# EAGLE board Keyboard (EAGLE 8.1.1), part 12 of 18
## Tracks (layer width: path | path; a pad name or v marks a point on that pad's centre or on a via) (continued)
S$12144 (continued)
  Bottom 0: 21.7,26.16 21.75,26.61
S$12145
  Bottom 0: 21.75,26.61 21.7,27.05
S$12146
  Bottom 0: 21.7,27.05 21.57,27.48
S$12147
  Bottom 0: 21.57,27.48 21.36,27.88
S$12148
  Bottom 0: 21.36,27.88 21.08,28.22
S$12149
  Bottom 0: 21.08,28.22 20.73,28.51
S$12150
  Bottom 0: 20.73,28.51 20.34,28.72
S$12151
  Bottom 0: 20.34,28.72 19.91,28.85
S$12152
  Bottom 0: 19.91,28.85 19.46,28.89
S$12153
  Bottom 0: 19.46,28.89 19.02,28.85
S$12154
  Bottom 0: 19.02,28.85 18.59,28.72
S$12155
  Bottom 0: 18.59,28.72 18.19,28.51
S$12156
  Bottom 0: 18.19,28.51 17.85,28.22
S$12157
  Bottom 0: 17.85,28.22 17.56,27.88
S$12158
  Bottom 0: 17.56,27.88 17.35,27.48
S$12159
  Bottom 0: 17.35,27.48 17.22,27.05
S$12160
  Bottom 0: 17.22,27.05 17.18,26.61
S$12161
  Bottom 0: 17.18,26.61 17.22,26.16
S$12162
  Bottom 0: 17.22,26.16 17.35,25.73
S$12163
  Bottom 0: 17.35,25.73 17.56,25.34
S$12164
  Bottom 0: 17.56,25.34 17.85,24.99
S$12165
  Bottom 0: 17.85,24.99 18.19,24.71
S$12166
  Bottom 0: 18.19,24.71 18.59,24.49
S$12167
  Bottom 0: 18.59,24.49 19.02,24.37
S$12168
  Bottom 0: 19.02,24.37 19.46,24.32
S$12169
  Bottom 0: 297.8,13.28 297.8,13.52
S$12170
  Bottom 0: 297.8,13.52 297.79,13.59
S$12171
  Bottom 0: 297.79,13.59 297.75,13.66
S$12172
  Bottom 0: 297.75,13.66 297.69,13.72
S$12173
  Bottom 0: 297.69,13.72 297.62,13.76
S$12174
  Bottom 0: 297.62,13.76 297.54,13.77
S$12175
  Bottom 0: 297.54,13.77 296.47,13.77
S$12176
  Bottom 0: 296.47,13.77 296.47,13.89
S$12177
  Bottom 0: 296.47,13.89 296.45,13.95
S$12178
  Bottom 0: 296.45,13.95 296.45,14
S$12179
  Bottom 0: 296.45,14 296.42,14.06
S$12180
  Bottom 0: 296.42,14.06 296.4,14.12
S$12181
  Bottom 0: 296.4,14.12 296.37,14.15
S$12182
  Bottom 0: 296.37,14.15 296.34,14.2
S$12183
  Bottom 0: 296.34,14.2 295.3,15.25
S$12184
  Bottom 0: 295.3,15.25 295.31,15.27
S$12185
  Bottom 0: 295.31,15.27 295.44,15.57
S$12186
  Bottom 0: 295.44,15.57 295.49,15.89
S$12187
  Bottom 0: 295.49,15.89 295.44,16.21
S$12188
  Bottom 0: 295.44,16.21 295.31,16.51
S$12189
  Bottom 0: 295.31,16.51 295.11,16.76
S$12190
  Bottom 0: 295.11,16.76 294.84,16.95
S$12191
  Bottom 0: 294.84,16.95 294.53,17.06
S$12192
  Bottom 0: 294.53,17.06 294.21,17.08
S$12193
  Bottom 0: 294.21,17.08 293.89,17.01
S$12194
  Bottom 0: 293.89,17.01 293.79,16.96
S$12195
  Bottom 0: 293.79,16.96 298.48,21.65
S$12196
  Bottom 0: 298.48,21.65 298.52,21.7
S$12197
  Bottom 0: 298.52,21.7 298.56,21.77
S$12198
  Bottom 0: 298.56,21.77 298.58,21.83
S$12199
  Bottom 0: 298.58,21.83 298.6,21.89
S$12200
  Bottom 0: 298.6,21.89 298.6,21.96
S$12201
  Bottom 0: 298.6,21.96 298.6,23.13
S$12202
  Bottom 0: 298.6,23.13 299.73,24.25
S$12203
  Bottom 0: 299.73,24.25 299.72,24.22
S$12204
  Bottom 0: 299.72,24.22 299.72,23.87
S$12205
  Bottom 0: 299.72,23.87 299.8,23.53
S$12206
  Bottom 0: 299.8,23.53 299.98,23.22
S$12207
  Bottom 0: 299.98,23.22 300.14,23.05
S$12208
  Bottom 0: 300.14,23.05 300.14,13.41
S$12209
  Bottom 0: 300.14,13.41 300.07,13.48
S$12210
  Bottom 0: 300.07,13.48 299.8,13.66
S$12211
  Bottom 0: 299.8,13.66 299.49,13.75
S$12212
  Bottom 0: 299.49,13.75 299.16,13.75
S$12213
  Bottom 0: 299.16,13.75 298.85,13.66
S$12214
  Bottom 0: 298.85,13.66 298.76,13.61
S$12215
  Bottom 0: 298.76,13.61 298.64,13.63
S$12216
  Bottom 0: 298.64,13.63 298.34,13.61
S$12217
  Bottom 0: 298.34,13.61 298.06,13.5
S$12218
  Bottom 0: 298.06,13.5 297.82,13.31
S$12219
  Bottom 0: 297.82,13.31 297.8,13.28
S$12220
  Bottom 0: 301.02,16.68 301.02,22.66
S$12221
  Bottom 0: 301.02,22.66 301.19,22.65
S$12222
  Bottom 0: 301.19,22.65 301.5,22.71
S$12223
  Bottom 0: 301.5,22.71 301.6,22.68
S$12224
  Bottom 0: 301.6,22.68 301.95,22.65
S$12225
  Bottom 0: 301.95,22.65 302.3,22.71
S$12226
  Bottom 0: 302.3,22.71 302.61,22.87
S$12227
  Bottom 0: 302.61,22.87 302.88,23.09
S$12228
  Bottom 0: 302.88,23.09 302.95,23.18
S$12229
  Bottom 0: 302.95,23.18 302.95,17.73
S$12230
  Bottom 0: 302.95,17.73 302.24,17.03
S$12231
  Bottom 0: 302.24,17.03 302.15,17.06
S$12232
  Bottom 0: 302.15,17.06 301.83,17.08
S$12233
  Bottom 0: 301.83,17.08 301.51,17.01
S$12234
  Bottom 0: 301.51,17.01 301.22,16.86
S$12235
  Bottom 0: 301.22,16.86 301.02,16.68
S$12236
  Bottom 0: 35.25,17.97 21.84,31.39
S$12237
  Bottom 0: 21.84,31.39 21.88,31.69
S$12238
  Bottom 0: 21.88,31.69 21.83,32.01
S$12239
  Bottom 0: 21.83,32.01 21.69,32.31
S$12240
  Bottom 0: 21.69,32.31 21.48,32.55
S$12241
  Bottom 0: 21.48,32.55 21.21,32.73
S$12242
  Bottom 0: 21.21,32.73 20.89,32.82
S$12243
  Bottom 0: 20.89,32.82 20.57,32.82
S$12244
  Bottom 0: 20.57,32.82 20.26,32.73
S$12245
  Bottom 0: 20.26,32.73 19.99,32.55
S$12246
  Bottom 0: 19.99,32.55 19.89,32.44
S$12247
  Bottom 0: 19.89,32.44 19.89,34.34
S$12248
  Bottom 0: 19.89,34.34 21.74,36.19
S$12249
  Bottom 0: 21.74,36.19 21.78,36.24
S$12250
  Bottom 0: 21.78,36.24 21.82,36.3
S$12251
  Bottom 0: 21.82,36.3 21.85,36.37
S$12252
  Bottom 0: 21.85,36.37 21.86,36.43
S$12253
  Bottom 0: 21.86,36.43 21.87,36.5
S$12254
  Bottom 0: 21.87,36.5 21.87,56.2
S$12255
  Bottom 0: 21.87,56.2 23.36,57.69
S$12256
  Bottom 0: 23.36,57.69 23.4,57.74
S$12257
  Bottom 0: 23.4,57.74 23.44,57.8
S$12258
  Bottom 0: 23.44,57.8 23.47,57.86
S$12259
  Bottom 0: 23.47,57.86 23.49,57.93
S$12260
  Bottom 0: 23.49,57.93 23.49,58
S$12261
  Bottom 0: 23.49,58 23.49,62.41
S$12262
  Bottom 0: 23.49,62.41 29.8,62.41
S$12263
  Bottom 0: 29.8,62.41 29.9,62.3
S$12264
  Bottom 0: 29.9,62.3 30.12,62.19
S$12265
  Bottom 0: 30.12,62.19 30.37,62.17
S$12266
  Bottom 0: 30.37,62.17 30.61,62.23
S$12267
  Bottom 0: 30.61,62.23 30.71,62.3
S$12268
  Bottom 0: 30.71,62.3 30.79,62.2
S$12269
  Bottom 0: 30.79,62.2 30.98,62
S$12270
  Bottom 0: 30.98,62 31.04,61.95
S$12271
  Bottom 0: 31.04,61.95 31.1,61.92
S$12272
  Bottom 0: 31.1,61.92 31.16,61.89
S$12273
  Bottom 0: 31.16,61.89 31.23,61.87
S$12274
  Bottom 0: 31.23,61.87 31.3,61.86
S$12275
  Bottom 0: 31.3,61.86 32.88,61.86
S$12276
  Bottom 0: 32.88,61.86 33.73,61.01
S$12277
  Bottom 0: 33.73,61.01 33.67,61.02
S$12278
  Bottom 0: 33.67,61.02 33.33,61
S$12279
  Bottom 0: 33.33,61 33,60.89
S$12280
  Bottom 0: 33,60.89 32.97,60.87
S$12281
  Bottom 0: 32.97,60.87 32.4,61.45
S$12282
  Bottom 0: 32.4,61.45 32.34,61.49
S$12283
  Bottom 0: 32.34,61.49 32.28,61.53
S$12284
  Bottom 0: 32.28,61.53 32.22,61.56
S$12285
  Bottom 0: 32.22,61.56 32.15,61.57
S$12286
  Bottom 0: 32.15,61.57 32.08,61.58
S$12287
  Bottom 0: 32.08,61.58 27.51,61.58
S$12288
  Bottom 0: 27.51,61.58 27.45,61.71
S$12289
  Bottom 0: 27.45,61.71 27.24,61.92
S$12290
  Bottom 0: 27.24,61.92 26.98,62.08
S$12291
  Bottom 0: 26.98,62.08 26.68,62.14
S$12292
  Bottom 0: 26.68,62.14 26.38,62.13
S$12293
  Bottom 0: 26.38,62.13 26.1,62.01
S$12294
  Bottom 0: 26.1,62.01 25.86,61.83
S$12295
  Bottom 0: 25.86,61.83 25.69,61.58
S$12296
  Bottom 0: 25.69,61.58 25.6,61.29
S$12297
  Bottom 0: 25.6,61.29 25.6,60.98
S$12298
  Bottom 0: 25.6,60.98 25.69,60.69
S$12299
  Bottom 0: 25.69,60.69 25.86,60.44
S$12300
  Bottom 0: 25.86,60.44 26.1,60.26
S$12301
  Bottom 0: 26.1,60.26 26.38,60.15
S$12302
  Bottom 0: 26.38,60.15 26.68,60.12
S$12303
  Bottom 0: 26.68,60.12 26.98,60.19
S$12304
  Bottom 0: 26.98,60.19 27.24,60.34
S$12305
  Bottom 0: 27.24,60.34 27.45,60.56
S$12306
  Bottom 0: 27.45,60.56 27.51,60.69
S$12307
  Bottom 0: 27.51,60.69 31.89,60.69
S$12308
  Bottom 0: 31.89,60.69 32.35,60.24
S$12309
  Bottom 0: 32.35,60.24 32.29,60.14
S$12310
  Bottom 0: 32.29,60.14 32.2,59.8
S$12311
  Bottom 0: 32.2,59.8 32.2,59.45
S$12312
  Bottom 0: 32.2,59.45 32.29,59.11
S$12313
  Bottom 0: 32.29,59.11 32.46,58.8
S$12314
  Bottom 0: 32.46,58.8 32.7,58.55
S$12315
  Bottom 0: 32.7,58.55 33,58.36
S$12316
  Bottom 0: 33,58.36 33.33,58.26
S$12317
  Bottom 0: 33.33,58.26 33.67,58.23
S$12318
  Bottom 0: 33.67,58.23 34.02,58.3
S$12319
  Bottom 0: 34.02,58.3 34.34,58.45
S$12320
  Bottom 0: 34.34,58.45 34.61,58.67
S$12321
  Bottom 0: 34.61,58.67 34.82,58.96
S$12322
  Bottom 0: 34.82,58.96 34.94,59.28
S$12323
  Bottom 0: 34.94,59.28 34.99,59.63
S$12324
  Bottom 0: 34.99,59.63 34.97,59.77
S$12325
  Bottom 0: 34.97,59.77 40.55,54.18
S$12326
  Bottom 0: 40.55,54.18 40.54,54.17
S$12327
  Bottom 0: 40.54,54.17 40.51,54.1
S$12328
  Bottom 0: 40.51,54.1 40.48,54.04
S$12329
  Bottom 0: 40.48,54.04 40.46,53.97
S$12330
  Bottom 0: 40.46,53.97 40.45,53.9
S$12331
  Bottom 0: 40.45,53.9 40.45,51.88
S$12332
  Bottom 0: 40.45,51.88 40.06,51.88
S$12333
  Bottom 0: 40.06,51.88 40.06,52.01
S$12334
  Bottom 0: 40.06,52.01 40,52.23
S$12335
  Bottom 0: 40,52.23 39.84,52.39
S$12336
  Bottom 0: 39.84,52.39 39.62,52.45
S$12337
  Bottom 0: 39.62,52.45 39.26,52.45
S$12338
  Bottom 0: 39.26,52.45 38.17,53.54
S$12339
  Bottom 0: 38.17,53.54 38.23,53.67
S$12340
  Bottom 0: 38.23,53.67 38.28,53.99
S$12341
  Bottom 0: 38.28,53.99 38.23,54.31
S$12342
  Bottom 0: 38.23,54.31 38.1,54.61
S$12343
  Bottom 0: 38.1,54.61 37.9,54.87
S$12344
  Bottom 0: 37.9,54.87 37.63,55.05
S$12345
  Bottom 0: 37.63,55.05 37.33,55.16
S$12346
  Bottom 0: 37.33,55.16 37.01,55.18
S$12347
  Bottom 0: 37.01,55.18 36.68,55.12
S$12348
  Bottom 0: 36.68,55.12 36.39,54.97
S$12349
  Bottom 0: 36.39,54.97 36.16,54.74
S$12350
  Bottom 0: 36.16,54.74 35.99,54.47
S$12351
  Bottom 0: 35.99,54.47 35.9,54.16
S$12352
  Bottom 0: 35.9,54.16 35.9,53.83
S$12353
  Bottom 0: 35.9,53.83 35.99,53.52
S$12354
  Bottom 0: 35.99,53.52 36.16,53.24
S$12355
  Bottom 0: 36.16,53.24 36.39,53.02
S$12356
  Bottom 0: 36.39,53.02 36.68,52.87
S$12357
  Bottom 0: 36.68,52.87 37.01,52.8
S$12358
  Bottom 0: 37.01,52.8 37.33,52.82
S$12359
  Bottom 0: 37.33,52.82 37.55,52.9
S$12360
  Bottom 0: 37.55,52.9 38.6,51.84
S$12361
  Bottom 0: 38.6,51.84 38.58,51.83
S$12362
  Bottom 0: 38.58,51.83 38.53,51.77
S$12363
  Bottom 0: 38.53,51.77 38.49,51.7
S$12364
  Bottom 0: 38.49,51.7 38.48,51.63
S$12365
  Bottom 0: 38.48,51.63 38.48,49.85
S$12366
  Bottom 0: 38.48,49.85 38.49,49.77
S$12367
  Bottom 0: 38.49,49.77 38.53,49.7
S$12368
  Bottom 0: 38.53,49.7 38.58,49.64
S$12369
  Bottom 0: 38.58,49.64 38.66,49.6
S$12370
  Bottom 0: 38.66,49.6 38.73,49.59
S$12371
  Bottom 0: 38.73,49.59 40.45,49.59
S$12372
  Bottom 0: 40.45,49.59 40.45,49.29
S$12373
  Bottom 0: 40.45,49.29 36.52,45.35
S$12374
  Bottom 0: 36.52,45.35 36.48,45.3
S$12375
  Bottom 0: 36.48,45.3 36.44,45.24
S$12376
  Bottom 0: 36.44,45.24 36.42,45.18
S$12377
  Bottom 0: 36.42,45.18 36.4,45.11
S$12378
  Bottom 0: 36.4,45.11 36.39,45.04
S$12379
  Bottom 0: 36.39,45.04 36.39,39.85
S$12380
  Bottom 0: 36.39,39.85 36.4,39.78
S$12381
  Bottom 0: 36.4,39.78 36.42,39.71
S$12382
  Bottom 0: 36.42,39.71 36.44,39.65
S$12383
  Bottom 0: 36.44,39.65 36.48,39.59
S$12384
  Bottom 0: 36.48,39.59 36.52,39.53
S$12385
  Bottom 0: 36.52,39.53 46.43,29.62
S$12386
  Bottom 0: 46.43,29.62 46.49,29.58
S$12387
  Bottom 0: 46.49,29.58 46.55,29.54
S$12388
  Bottom 0: 46.55,29.54 46.61,29.52
S$12389
  Bottom 0: 46.61,29.52 46.68,29.5
S$12390
  Bottom 0: 46.68,29.5 46.75,29.5
S$12391
  Bottom 0: 46.75,29.5 50.3,29.5
S$12392
  Bottom 0: 50.3,29.5 51,28.81
S$12393
  Bottom 0: 51,28.81 50.86,28.85
S$12394
  Bottom 0: 50.86,28.85 50.42,28.89
S$12395
  Bottom 0: 50.42,28.89 49.97,28.85
S$12396
  Bottom 0: 49.97,28.85 49.54,28.72
S$12397
  Bottom 0: 49.54,28.72 49.15,28.51
S$12398
  Bottom 0: 49.15,28.51 48.8,28.22
S$12399
  Bottom 0: 48.8,28.22 48.52,27.88
S$12400
  Bottom 0: 48.52,27.88 48.3,27.48
S$12401
  Bottom 0: 48.3,27.48 48.17,27.05
S$12402
  Bottom 0: 48.17,27.05 48.13,26.61
S$12403
  Bottom 0: 48.13,26.61 48.17,26.16
S$12404
  Bottom 0: 48.17,26.16 48.3,25.73
S$12405
  Bottom 0: 48.3,25.73 48.52,25.34
S$12406
  Bottom 0: 48.52,25.34 48.8,24.99
S$12407
  Bottom 0: 48.8,24.99 49.15,24.71
S$12408
  Bottom 0: 49.15,24.71 49.54,24.49
S$12409
  Bottom 0: 49.54,24.49 49.97,24.37
S$12410
  Bottom 0: 49.97,24.37 50.42,24.32
S$12411
  Bottom 0: 50.42,24.32 50.86,24.37
S$12412
  Bottom 0: 50.86,24.37 51.29,24.49
S$12413
  Bottom 0: 51.29,24.49 51.69,24.71
S$12414
  Bottom 0: 51.69,24.71 52.03,24.99
S$12415
  Bottom 0: 52.03,24.99 52.32,25.34
S$12416
  Bottom 0: 52.32,25.34 52.53,25.73
S$12417
  Bottom 0: 52.53,25.73 52.65,26.16
S$12418
  Bottom 0: 52.65,26.16 52.7,26.61
S$12419
  Bottom 0: 52.7,26.61 52.65,27.05
S$12420
  Bottom 0: 52.65,27.05 52.61,27.19
S$12421
  Bottom 0: 52.61,27.19 53.78,26.02
S$12422
  Bottom 0: 53.78,26.02 53.78,25.38
S$12423
  Bottom 0: 53.78,25.38 53.63,25.33
S$12424
  Bottom 0: 53.63,25.33 53.34,25.14
S$12425
  Bottom 0: 53.34,25.14 53.1,24.89
S$12426
  Bottom 0: 53.1,24.89 52.93,24.58
S$12427
  Bottom 0: 52.93,24.58 52.84,24.24
S$12428
  Bottom 0: 52.84,24.24 52.84,23.89
S$12429
  Bottom 0: 52.84,23.89 52.93,23.55
S$12430
  Bottom 0: 52.93,23.55 53.1,23.24
S$12431
  Bottom 0: 53.1,23.24 53.34,22.99
S$12432
  Bottom 0: 53.34,22.99 53.63,22.8
S$12433
  Bottom 0: 53.63,22.8 53.96,22.7
S$12434
  Bottom 0: 53.96,22.7 54.31,22.68
S$12435
  Bottom 0: 54.31,22.68 54.66,22.74
S$12436
  Bottom 0: 54.66,22.74 54.97,22.89
S$12437
  Bottom 0: 54.97,22.89 55.24,23.11
S$12438
  Bottom 0: 55.24,23.11 55.42,23.36
S$12439
  Bottom 0: 55.42,23.36 55.42,17.97
S$12440
  Bottom 0: 55.42,17.97 35.25,17.97
S$12441
  Bottom 0: 47.96,20.14 48.31,20.2
S$12442
  Bottom 0: 48.31,20.2 48.62,20.35
S$12443
  Bottom 0: 48.62,20.35 48.89,20.57
S$12444
  Bottom 0: 48.89,20.57 49.1,20.86
S$12445
  Bottom 0: 49.1,20.86 49.23,21.18
S$12446
  Bottom 0: 49.23,21.18 49.27,21.53
S$12447
  Bottom 0: 49.27,21.53 49.23,21.87
S$12448
  Bottom 0: 49.23,21.87 49.1,22.2
S$12449
  Bottom 0: 49.1,22.2 48.89,22.48
S$12450
  Bottom 0: 48.89,22.48 48.62,22.7
S$12451
  Bottom 0: 48.62,22.7 48.31,22.86
S$12452
  Bottom 0: 48.31,22.86 47.96,22.92
S$12453
  Bottom 0: 47.96,22.92 47.61,22.9
S$12454
  Bottom 0: 47.61,22.9 47.28,22.79
S$12455
  Bottom 0: 47.28,22.79 47.25,22.78
S$12456
  Bottom 0: 47.25,22.78 46.69,23.34
S$12457
  Bottom 0: 46.69,23.34 46.64,23.39
S$12458
  Bottom 0: 46.64,23.39 46.58,23.42
S$12459
  Bottom 0: 46.58,23.42 46.52,23.45
S$12460
  Bottom 0: 46.52,23.45 46.45,23.47
S$12461
  Bottom 0: 46.45,23.47 46.38,23.47
S$12462
  Bottom 0: 46.38,23.47 42.99,23.47
S$12463
  Bottom 0: 42.99,23.47 42.93,23.6
S$12464
  Bottom 0: 42.93,23.6 42.73,23.82
S$12465
  Bottom 0: 42.73,23.82 42.46,23.98
S$12466
  Bottom 0: 42.46,23.98 42.17,24.04
S$12467
  Bottom 0: 42.17,24.04 41.86,24.02
S$12468
  Bottom 0: 41.86,24.02 41.58,23.91
S$12469
  Bottom 0: 41.58,23.91 41.34,23.72
S$12470
  Bottom 0: 41.34,23.72 41.18,23.47
S$12471
  Bottom 0: 41.18,23.47 41.08,23.18
S$12472
  Bottom 0: 41.08,23.18 41.08,22.88
S$12473
  Bottom 0: 41.08,22.88 41.18,22.59
S$12474
  Bottom 0: 41.18,22.59 41.34,22.34
S$12475
  Bottom 0: 41.34,22.34 41.58,22.15
S$12476
  Bottom 0: 41.58,22.15 41.86,22.04
S$12477
  Bottom 0: 41.86,22.04 42.17,22.02
S$12478
  Bottom 0: 42.17,22.02 42.46,22.09
S$12479
  Bottom 0: 42.46,22.09 42.73,22.24
S$12480
  Bottom 0: 42.73,22.24 42.93,22.46
S$12481
  Bottom 0: 42.93,22.46 42.99,22.59
S$12482
  Bottom 0: 42.99,22.59 46.2,22.59
S$12483
  Bottom 0: 46.2,22.59 46.64,22.15
S$12484
  Bottom 0: 46.64,22.15 46.58,22.04
S$12485
  Bottom 0: 46.58,22.04 46.49,21.7
S$12486
  Bottom 0: 46.49,21.7 46.49,21.35
S$12487
  Bottom 0: 46.49,21.35 46.58,21.01
S$12488
  Bottom 0: 46.58,21.01 46.75,20.7
S$12489
  Bottom 0: 46.75,20.7 46.99,20.45
S$12490
  Bottom 0: 46.99,20.45 47.28,20.26
S$12491
  Bottom 0: 47.28,20.26 47.61,20.16
S$12492
  Bottom 0: 47.61,20.16 47.96,20.14
S$12493
  Bottom 0: 39.78,22.02 40.08,22.09
S$12494
  Bottom 0: 40.08,22.09 40.34,22.24
S$12495
  Bottom 0: 40.34,22.24 40.55,22.46
S$12496
  Bottom 0: 40.55,22.46 40.68,22.74
S$12497
  Bottom 0: 40.68,22.74 40.72,23.04
S$12498
  Bottom 0: 40.72,23.04 40.68,23.34
S$12499
  Bottom 0: 40.68,23.34 40.55,23.61
S$12500
  Bottom 0: 40.55,23.61 40.34,23.83
S$12501
  Bottom 0: 40.34,23.83 40.08,23.98
S$12502
  Bottom 0: 40.08,23.98 39.78,24.05
S$12503
  Bottom 0: 39.78,24.05 39.48,24.03
S$12504
  Bottom 0: 39.48,24.03 39.2,23.91
S$12505
  Bottom 0: 39.2,23.91 38.96,23.73
S$12506
  Bottom 0: 38.96,23.73 38.79,23.48
S$12507
  Bottom 0: 38.79,23.48 38.7,23.19
S$12508
  Bottom 0: 38.7,23.19 38.7,22.88
S$12509
  Bottom 0: 38.7,22.88 38.79,22.59
S$12510
  Bottom 0: 38.79,22.59 38.96,22.34
S$12511
  Bottom 0: 38.96,22.34 39.2,22.16
S$12512
  Bottom 0: 39.2,22.16 39.48,22.05
S$12513
  Bottom 0: 39.48,22.05 39.78,22.02
S$12514
  Bottom 0: 42.17,29.64 42.46,29.7
S$12515
  Bottom 0: 42.46,29.7 42.73,29.86
S$12516
  Bottom 0: 42.73,29.86 42.93,30.08
S$12517
  Bottom 0: 42.93,30.08 43.06,30.35
S$12518
  Bottom 0: 43.06,30.35 43.11,30.65
S$12519
  Bottom 0: 43.11,30.65 43.06,30.95
S$12520
  Bottom 0: 43.06,30.95 42.93,31.22
S$12521
  Bottom 0: 42.93,31.22 42.73,31.44
S$12522
  Bottom 0: 42.73,31.44 42.46,31.59
S$12523
  Bottom 0: 42.46,31.59 42.17,31.66
S$12524
  Bottom 0: 42.17,31.66 41.86,31.64
S$12525
  Bottom 0: 41.86,31.64 41.58,31.53
S$12526
  Bottom 0: 41.58,31.53 41.34,31.34
S$12527
  Bottom 0: 41.34,31.34 41.18,31.09
S$12528
  Bottom 0: 41.18,31.09 41.08,30.8
S$12529
  Bottom 0: 41.08,30.8 41.08,30.5
S$12530
  Bottom 0: 41.08,30.5 41.18,30.21
S$12531
  Bottom 0: 41.18,30.21 41.34,29.96
S$12532
  Bottom 0: 41.34,29.96 41.58,29.77
S$12533
  Bottom 0: 41.58,29.77 41.86,29.66
S$12534
  Bottom 0: 41.86,29.66 42.17,29.64
S$12535
  Bottom 0: 39.78,29.64 40.08,29.71
S$12536
  Bottom 0: 40.08,29.71 40.34,29.86
S$12537
  Bottom 0: 40.34,29.86 40.55,30.08
S$12538
  Bottom 0: 40.55,30.08 40.68,30.36
S$12539
  Bottom 0: 40.68,30.36 40.72,30.66
S$12540
  Bottom 0: 40.72,30.66 40.68,30.95
S$12541
  Bottom 0: 40.68,30.95 40.55,31.23
S$12542
  Bottom 0: 40.55,31.23 40.34,31.45
S$12543
  Bottom 0: 40.34,31.45 40.08,31.6
S$12544
  Bottom 0: 40.08,31.6 39.78,31.67
S$12545
  Bottom 0: 39.78,31.67 39.48,31.65
S$12546
  Bottom 0: 39.48,31.65 39.2,31.53
S$12547
  Bottom 0: 39.2,31.53 38.96,31.35
S$12548
  Bottom 0: 38.96,31.35 38.79,31.1
S$12549
  Bottom 0: 38.79,31.1 38.7,30.81
S$12550
  Bottom 0: 38.7,30.81 38.7,30.5
S$12551
  Bottom 0: 38.7,30.5 38.79,30.21
S$12552
  Bottom 0: 38.79,30.21 38.96,29.96
S$12553
  Bottom 0: 38.96,29.96 39.2,29.78
S$12554
  Bottom 0: 39.2,29.78 39.48,29.66
S$12555
  Bottom 0: 39.48,29.66 39.78,29.64
S$12556
  Bottom 0: 32.64,35.12 32.94,35.18
S$12557
  Bottom 0: 32.94,35.18 33.2,35.33
S$12558
  Bottom 0: 33.2,35.33 33.4,35.55
S$12559
  Bottom 0: 33.4,35.55 33.53,35.83
S$12560
  Bottom 0: 33.53,35.83 33.58,36.13
S$12561
  Bottom 0: 33.58,36.13 33.53,36.43
S$12562
  Bottom 0: 33.53,36.43 33.4,36.7
S$12563
  Bottom 0: 33.4,36.7 33.2,36.92
S$12564
  Bottom 0: 33.2,36.92 32.94,37.07
S$12565
  Bottom 0: 32.94,37.07 32.64,37.14
S$12566
  Bottom 0: 32.64,37.14 32.34,37.12
S$12567
  Bottom 0: 32.34,37.12 32.05,37.01
S$12568
  Bottom 0: 32.05,37.01 31.82,36.82
S$12569
  Bottom 0: 31.82,36.82 31.65,36.57
S$12570
  Bottom 0: 31.65,36.57 31.56,36.28
S$12571
  Bottom 0: 31.56,36.28 31.56,35.97
S$12572
  Bottom 0: 31.56,35.97 31.65,35.68
S$12573
  Bottom 0: 31.65,35.68 31.82,35.44
S$12574
  Bottom 0: 31.82,35.44 32.05,35.25
S$12575
  Bottom 0: 32.05,35.25 32.34,35.14
S$12576
  Bottom 0: 32.34,35.14 32.64,35.12
S$12577
  Bottom 0: 23.11,35.12 23.4,35.18
S$12578
  Bottom 0: 23.4,35.18 23.67,35.33
S$12579
  Bottom 0: 23.67,35.33 23.87,35.55
S$12580
  Bottom 0: 23.87,35.55 24.01,35.83
S$12581
  Bottom 0: 24.01,35.83 24.05,36.13
S$12582
  Bottom 0: 24.05,36.13 24.01,36.43
S$12583
  Bottom 0: 24.01,36.43 23.87,36.7
S$12584
  Bottom 0: 23.87,36.7 23.67,36.92
S$12585
  Bottom 0: 23.67,36.92 23.4,37.07
S$12586
  Bottom 0: 23.4,37.07 23.11,37.14
S$12587
  Bottom 0: 23.11,37.14 22.81,37.12
S$12588
  Bottom 0: 22.81,37.12 22.53,37.01
S$12589
  Bottom 0: 22.53,37.01 22.29,36.82
S$12590
  Bottom 0: 22.29,36.82 22.12,36.57
S$12591
  Bottom 0: 22.12,36.57 22.03,36.28
S$12592
  Bottom 0: 22.03,36.28 22.03,35.97
S$12593
  Bottom 0: 22.03,35.97 22.12,35.68
S$12594
  Bottom 0: 22.12,35.68 22.29,35.44
S$12595
  Bottom 0: 22.29,35.44 22.53,35.25
S$12596
  Bottom 0: 22.53,35.25 22.81,35.14
S$12597
  Bottom 0: 22.81,35.14 23.11,35.12
S$12598
  Bottom 0: 32.64,42.74 32.94,42.8
S$12599
  Bottom 0: 32.94,42.8 33.2,42.95
S$12600
  Bottom 0: 33.2,42.95 33.4,43.17
S$12601
  Bottom 0: 33.4,43.17 33.53,43.44
S$12602
  Bottom 0: 33.53,43.44 33.58,43.75
S$12603
  Bottom 0: 33.58,43.75 33.53,44.05
S$12604
  Bottom 0: 33.53,44.05 33.4,44.32
S$12605
  Bottom 0: 33.4,44.32 33.2,44.54
S$12606
  Bottom 0: 33.2,44.54 32.94,44.69
S$12607
  Bottom 0: 32.94,44.69 32.64,44.76
S$12608
  Bottom 0: 32.64,44.76 32.34,44.74
S$12609
  Bottom 0: 32.34,44.74 32.05,44.62
S$12610
  Bottom 0: 32.05,44.62 31.82,44.44
S$12611
  Bottom 0: 31.82,44.44 31.65,44.19
S$12612
  Bottom 0: 31.65,44.19 31.56,43.9
S$12613
  Bottom 0: 31.56,43.9 31.56,43.59
S$12614
  Bottom 0: 31.56,43.59 31.65,43.3
S$12615
  Bottom 0: 31.65,43.3 31.82,43.06
S$12616
  Bottom 0: 31.82,43.06 32.05,42.87
S$12617
  Bottom 0: 32.05,42.87 32.34,42.75
S$12618
  Bottom 0: 32.34,42.75 32.64,42.74
S$12619
  Bottom 0: 23.11,42.74 23.4,42.8
S$12620
  Bottom 0: 23.4,42.8 23.67,42.95
S$12621
  Bottom 0: 23.67,42.95 23.87,43.17
S$12622
  Bottom 0: 23.87,43.17 24.01,43.44
S$12623
  Bottom 0: 24.01,43.44 24.05,43.75
S$12624
  Bottom 0: 24.05,43.75 24.01,44.05
S$12625
  Bottom 0: 24.01,44.05 23.87,44.32
S$12626
  Bottom 0: 23.87,44.32 23.67,44.54
S$12627
  Bottom 0: 23.67,44.54 23.4,44.69
S$12628
  Bottom 0: 23.4,44.69 23.11,44.76
S$12629
  Bottom 0: 23.11,44.76 22.81,44.74
S$12630
  Bottom 0: 22.81,44.74 22.53,44.62
S$12631
  Bottom 0: 22.53,44.62 22.29,44.44
S$12632
  Bottom 0: 22.29,44.44 22.12,44.19
S$12633
  Bottom 0: 22.12,44.19 22.03,43.9
S$12634
  Bottom 0: 22.03,43.9 22.03,43.59
S$12635
  Bottom 0: 22.03,43.59 22.12,43.3
S$12636
  Bottom 0: 22.12,43.3 22.29,43.06
S$12637
  Bottom 0: 22.29,43.06 22.53,42.87
S$12638
  Bottom 0: 22.53,42.87 22.81,42.75
S$12639
  Bottom 0: 22.81,42.75 23.11,42.74
S$12640
  Bottom 0: 29.33,43.59 29.68,43.79
S$12641
  Bottom 0: 29.68,43.79 30.09,44.13
S$12642
  Bottom 0: 30.09,44.13 30.45,44.53
S$12643
  Bottom 0: 30.45,44.53 30.73,44.97
S$12644
  Bottom 0: 30.73,44.97 30.74,44.99
S$12645
  Bottom 0: 30.74,44.99 29.33,44.99
S$12646
  Bottom 0: 29.33,44.99 29.33,43.59
S$12647
  Bottom 0: 26.28,43.59 26.28,44.99
S$12648
  Bottom 0: 26.28,44.99 24.89,44.99
S$12649
  Bottom 0: 24.89,44.99 25.02,44.75
S$12650
  Bottom 0: 25.02,44.75 25.33,44.32
S$12651
  Bottom 0: 25.33,44.32 25.72,43.95
S$12652
  Bottom 0: 25.72,43.95 26.15,43.65
S$12653
  Bottom 0: 26.15,43.65 26.28,43.59
S$12654
  Bottom 0: 29.33,48.03 30.74,48.03
S$12655
  Bottom 0: 30.74,48.03 30.73,48.04
S$12656
  Bottom 0: 30.73,48.04 30.45,48.49
S$12657
  Bottom 0: 30.45,48.49 30.09,48.89
S$12658
  Bottom 0: 30.09,48.89 29.68,49.23
S$12659
  Bottom 0: 29.68,49.23 29.33,49.43
S$12660
  Bottom 0: 29.33,49.43 29.33,48.03
S$12661
  Bottom 0: 24.89,48.03 26.28,48.03
S$12662
  Bottom 0: 26.28,48.03 26.28,49.43
S$12663
  Bottom 0: 26.28,49.43 26.15,49.37
S$12664
  Bottom 0: 26.15,49.37 25.72,49.06
S$12665
  Bottom 0: 25.72,49.06 25.33,48.7
S$12666
  Bottom 0: 25.33,48.7 25.02,48.27
S$12667
  Bottom 0: 25.02,48.27 24.89,48.03
S$12668
  Bottom 0: 148.29,20.34 148.29,23.34
S$12669
  Bottom 0: 148.29,23.34 148.35,23.24
S$12670
  Bottom 0: 148.35,23.24 148.59,22.99
S$12671
  Bottom 0: 148.59,22.99 148.88,22.8
S$12672
  Bottom 0: 148.88,22.8 149.21,22.7
S$12673
  Bottom 0: 149.21,22.7 149.56,22.68
S$12674
  Bottom 0: 149.56,22.68 149.91,22.74
S$12675
  Bottom 0: 149.91,22.74 150.22,22.89
S$12676
  Bottom 0: 150.22,22.89 150.49,23.11
S$12677
  Bottom 0: 150.49,23.11 150.7,23.4
S$12678
  Bottom 0: 150.7,23.4 150.82,23.72
S$12679
  Bottom 0: 150.82,23.72 150.87,24.07
S$12680
  Bottom 0: 150.87,24.07 150.82,24.41
S$12681
  Bottom 0: 150.82,24.41 150.7,24.74
S$12682
  Bottom 0: 150.7,24.74 150.49,25.02
S$12683
  Bottom 0: 150.49,25.02 150.22,25.25
S$12684
  Bottom 0: 150.22,25.25 149.92,25.39
S$12685
  Bottom 0: 149.92,25.39 149.92,33.03
S$12686
  Bottom 0: 149.92,33.03 149.91,33.1
S$12687
  Bottom 0: 149.91,33.1 149.9,33.17
S$12688
  Bottom 0: 149.9,33.17 149.87,33.24
S$12689
  Bottom 0: 149.87,33.24 149.83,33.29
S$12690
  Bottom 0: 149.83,33.29 149.79,33.35
S$12691
  Bottom 0: 149.79,33.35 149.38,33.75
S$12692
  Bottom 0: 149.38,33.75 149.41,33.75
S$12693
  Bottom 0: 149.41,33.75 149.74,33.77
S$12694
  Bottom 0: 149.74,33.77 150.04,33.88
S$12695
  Bottom 0: 150.04,33.88 150.3,34.06
S$12696
  Bottom 0: 150.3,34.06 150.51,34.32
S$12697
  Bottom 0: 150.51,34.32 150.53,34.37
S$12698
  Bottom 0: 150.53,34.37 153.28,34.37
S$12699
  Bottom 0: 153.28,34.37 153.37,34.37
S$12700
  Bottom 0: 153.37,34.37 153.45,34.39
S$12701
  Bottom 0: 153.45,34.39 153.53,34.43
S$12702
  Bottom 0: 153.53,34.43 153.61,34.48
S$12703
  Bottom 0: 153.61,34.48 153.68,34.54
S$12704
  Bottom 0: 153.68,34.54 160.77,41.63
S$12705
  Bottom 0: 160.77,41.63 167.36,35.03
S$12706
  Bottom 0: 167.36,35.03 167.36,34.77
S$12707
  Bottom 0: 167.36,34.77 167.45,34.46
S$12708
  Bottom 0: 167.45,34.46 167.62,34.19
S$12709
  Bottom 0: 167.62,34.19 167.85,33.96
S$12710
  Bottom 0: 167.85,33.96 168.15,33.81
S$12711
  Bottom 0: 168.15,33.81 168.47,33.75
S$12712
  Bottom 0: 168.47,33.75 168.79,33.77
S$12713
  Bottom 0: 168.79,33.77 168.88,33.8
S$12714
  Bottom 0: 168.88,33.8 170.01,32.67
S$12715
  Bottom 0: 170.01,32.67 170.07,32.61
S$12716
  Bottom 0: 170.07,32.61 170.15,32.56
S$12717
  Bottom 0: 170.15,32.56 170.23,32.53
S$12718
  Bottom 0: 170.23,32.53 170.32,32.51
S$12719
  Bottom 0: 170.32,32.51 170.41,32.5
S$12720
  Bottom 0: 170.41,32.5 177.41,32.5
S$12721
  Bottom 0: 177.41,32.5 177.41,31.35
S$12722
  Bottom 0: 177.41,31.35 177.26,31.45
S$12723
  Bottom 0: 177.26,31.45 177.02,31.52
S$12724
  Bottom 0: 177.02,31.52 176.77,31.5
S$12725
  Bottom 0: 176.77,31.5 176.55,31.39
S$12726
  Bottom 0: 176.55,31.39 176.38,31.2
S$12727
  Bottom 0: 176.38,31.2 176.28,30.96
S$12728
  Bottom 0: 176.28,30.96 173.27,27.95
S$12729
  Bottom 0: 173.27,27.95 170.53,27.95
S$12730
  Bottom 0: 170.53,27.95 167.09,31.39
S$12731
  Bottom 0: 167.09,31.39 167.13,31.69
S$12732
  Bottom 0: 167.13,31.69 167.1,31.9
S$12733
  Bottom 0: 167.1,31.9 168.66,30.34
S$12734
  Bottom 0: 168.66,30.34 168.72,30.3
S$12735
  Bottom 0: 168.72,30.3 168.78,30.25
S$12736
  Bottom 0: 168.78,30.25 168.84,30.23
S$12737
  Bottom 0: 168.84,30.23 168.91,30.21
S$12738
  Bottom 0: 168.91,30.21 168.98,30.21
S$12739
  Bottom 0: 168.98,30.21 173.34,30.21
S$12740
  Bottom 0: 173.34,30.21 173.51,29.96
S$12741
  Bottom 0: 173.51,29.96 173.75,29.77
S$12742
  Bottom 0: 173.75,29.77 174.03,29.66
S$12743
  Bottom 0: 174.03,29.66 174.33,29.64
S$12744
  Bottom 0: 174.33,29.64 174.63,29.7
S$12745
  Bottom 0: 174.63,29.7 174.89,29.86
S$12746
  Bottom 0: 174.89,29.86 175.09,30.08
S$12747
  Bottom 0: 175.09,30.08 175.22,30.35
S$12748
  Bottom 0: 175.22,30.35 175.27,30.65
S$12749
  Bottom 0: 175.27,30.65 175.22,30.95
S$12750
  Bottom 0: 175.22,30.95 175.09,31.22
S$12751
  Bottom 0: 175.09,31.22 174.89,31.44
S$12752
  Bottom 0: 174.89,31.44 174.63,31.59
S$12753
  Bottom 0: 174.63,31.59 174.33,31.66
S$12754
  Bottom 0: 174.33,31.66 174.03,31.64
S$12755
  Bottom 0: 174.03,31.64 173.75,31.53
S$12756
  Bottom 0: 173.75,31.53 173.51,31.34
S$12757
  Bottom 0: 173.51,31.34 173.34,31.09
S$12758
  Bottom 0: 173.34,31.09 169.17,31.09
S$12759
  Bottom 0: 169.17,31.09 166.99,33.27
S$12760
  Bottom 0: 166.99,33.27 166.93,33.31
S$12761
  Bottom 0: 166.93,33.31 166.87,33.35
S$12762
  Bottom 0: 166.87,33.35 166.81,33.38
S$12763
  Bottom 0: 166.81,33.38 166.74,33.39
S$12764
  Bottom 0: 166.74,33.39 166.67,33.4
S$12765
  Bottom 0: 166.67,33.4 165.41,33.4
S$12766
  Bottom 0: 165.41,33.4 165.34,33.39
S$12767
  Bottom 0: 165.34,33.39 165.28,33.38
S$12768
  Bottom 0: 165.28,33.38 165.21,33.35
S$12769
  Bottom 0: 165.21,33.35 165.15,33.31
S$12770
  Bottom 0: 165.15,33.31 165.1,33.27
S$12771
  Bottom 0: 165.1,33.27 164.54,32.71
S$12772
  Bottom 0: 164.54,32.71 164.54,32.72
S$12773
  Bottom 0: 164.54,32.72 164.48,32.78
S$12774
  Bottom 0: 164.48,32.78 164.41,32.82
S$12775
  Bottom 0: 164.41,32.82 164.34,32.83
S$12776
  Bottom 0: 164.34,32.83 163.89,32.83
S$12777
  Bottom 0: 163.89,32.83 163.89,32.96
S$12778
  Bottom 0: 163.89,32.96 163.83,33.18
S$12779
  Bottom 0: 163.83,33.18 163.66,33.34
S$12780
  Bottom 0: 163.66,33.34 163.45,33.4
S$12781
  Bottom 0: 163.45,33.4 163.1,33.4
S$12782
  Bottom 0: 163.1,33.4 162.01,34.48
S$12783
  Bottom 0: 162.01,34.48 162.07,34.62
S$12784
  Bottom 0: 162.07,34.62 162.12,34.94
S$12785
  Bottom 0: 162.12,34.94 162.07,35.26
S$12786
  Bottom 0: 162.07,35.26 161.95,35.56
S$12787
  Bottom 0: 161.95,35.56 161.74,35.81
S$12788
  Bottom 0: 161.74,35.81 161.47,36
S$12789
  Bottom 0: 161.47,36 161.17,36.11
S$12790
  Bottom 0: 161.17,36.11 160.84,36.13
S$12791
  Bottom 0: 160.84,36.13 160.53,36.06
S$12792
  Bottom 0: 160.53,36.06 160.24,35.91
S$12793
  Bottom 0: 160.24,35.91 160,35.69
S$12794
  Bottom 0: 160,35.69 159.83,35.41
S$12795
  Bottom 0: 159.83,35.41 159.74,35.1
S$12796
  Bottom 0: 159.74,35.1 159.74,34.77
S$12797
  Bottom 0: 159.74,34.77 159.83,34.46
S$12798
  Bottom 0: 159.83,34.46 160,34.19
S$12799
  Bottom 0: 160,34.19 160.24,33.96
S$12800
  Bottom 0: 160.24,33.96 160.53,33.81
S$12801
  Bottom 0: 160.53,33.81 160.84,33.75
S$12802
  Bottom 0: 160.84,33.75 161.17,33.77
S$12803
  Bottom 0: 161.17,33.77 161.39,33.85
S$12804
  Bottom 0: 161.39,33.85 162.44,32.79
S$12805
  Bottom 0: 162.44,32.79 162.41,32.78
S$12806
  Bottom 0: 162.41,32.78 162.35,32.72
S$12807
  Bottom 0: 162.35,32.72 162.31,32.65
S$12808
  Bottom 0: 162.31,32.65 162.3,32.58
S$12809
  Bottom 0: 162.3,32.58 162.3,30.8
S$12810
  Bottom 0: 162.3,30.8 162.31,30.73
S$12811
  Bottom 0: 162.31,30.73 156.21,30.73
S$12812
  Bottom 0: 156.21,30.73 156.18,30.95
S$12813
  Bottom 0: 156.18,30.95 156.04,31.22
S$12814
  Bottom 0: 156.04,31.22 155.84,31.44
S$12815
  Bottom 0: 155.84,31.44 155.58,31.59
S$12816
  Bottom 0: 155.58,31.59 155.28,31.66
S$12817
  Bottom 0: 155.28,31.66 154.98,31.64
S$12818
  Bottom 0: 154.98,31.64 154.7,31.53
S$12819
  Bottom 0: 154.7,31.53 154.46,31.34
S$12820
  Bottom 0: 154.46,31.34 154.29,31.09
S$12821
  Bottom 0: 154.29,31.09 154.2,30.8
S$12822
  Bottom 0: 154.2,30.8 154.2,30.5
S$12823
  Bottom 0: 154.2,30.5 154.29,30.21
S$12824
  Bottom 0: 154.29,30.21 154.46,29.96
S$12825
  Bottom 0: 154.46,29.96 154.7,29.77
S$12826
  Bottom 0: 154.7,29.77 154.98,29.66
S$12827
  Bottom 0: 154.98,29.66 155.28,29.64
S$12828
  Bottom 0: 155.28,29.64 155.58,29.7
S$12829
  Bottom 0: 155.58,29.7 155.82,29.84
S$12830
  Bottom 0: 155.82,29.84 164.45,29.84
S$12831
  Bottom 0: 164.45,29.84 164.52,29.85
S$12832
  Bottom 0: 164.52,29.85 164.59,29.86
S$12833
  Bottom 0: 164.59,29.86 164.65,29.89
S$12834
  Bottom 0: 164.65,29.89 164.71,29.93
S$12835
  Bottom 0: 164.71,29.93 164.77,29.97
S$12836
  Bottom 0: 164.77,29.97 165.02,30.22
S$12837
  Bottom 0: 165.02,30.22 165.06,30.28
S$12838
  Bottom 0: 165.06,30.28 165.1,30.34
S$12839
  Bottom 0: 165.1,30.34 165.13,30.4
S$12840
  Bottom 0: 165.13,30.4 165.14,30.47
S$12841
  Bottom 0: 165.14,30.47 165.15,30.54
S$12842
  Bottom 0: 165.15,30.54 165.15,30.93
S$12843
  Bottom 0: 165.15,30.93 165.24,30.82
S$12844
  Bottom 0: 165.24,30.82 165.51,30.64
S$12845
  Bottom 0: 165.51,30.64 165.82,30.55
S$12846
  Bottom 0: 165.82,30.55 166.15,30.55
S$12847
  Bottom 0: 166.15,30.55 166.28,30.59
S$12848
  Bottom 0: 166.28,30.59 169.72,27.14
S$12849
  Bottom 0: 169.72,27.14 169.72,24.77
S$12850
  Bottom 0: 169.72,24.77 169.54,25.02
S$12851
  Bottom 0: 169.54,25.02 169.27,25.25
S$12852
  Bottom 0: 169.27,25.25 168.96,25.4
S$12853
  Bottom 0: 168.96,25.4 168.61,25.46
S$12854
  Bottom 0: 168.61,25.46 168.26,25.44
S$12855
  Bottom 0: 168.26,25.44 167.93,25.33
S$12856
  Bottom 0: 167.93,25.33 167.64,25.14
S$12857
  Bottom 0: 167.64,25.14 167.4,24.89
S$12858
  Bottom 0: 167.4,24.89 167.22,24.58
S$12859
  Bottom 0: 167.22,24.58 167.14,24.24
S$12860
  Bottom 0: 167.14,24.24 167.14,23.89
S$12861
  Bottom 0: 167.14,23.89 167.22,23.55
S$12862
  Bottom 0: 167.22,23.55 167.28,23.45
S$12863
  Bottom 0: 167.28,23.45 164.17,20.34
S$12864
  Bottom 0: 164.17,20.34 162.91,20.34
S$12865
  Bottom 0: 162.91,20.34 162.92,20.35
S$12866
  Bottom 0: 162.92,20.35 163.19,20.57
S$12867
  Bottom 0: 163.19,20.57 163.4,20.86
S$12868
  Bottom 0: 163.4,20.86 163.53,21.18
S$12869
  Bottom 0: 163.53,21.18 163.57,21.53
S$12870
  Bottom 0: 163.57,21.53 163.53,21.87
S$12871
  Bottom 0: 163.53,21.87 163.4,22.2
S$12872
  Bottom 0: 163.4,22.2 163.19,22.48
S$12873
  Bottom 0: 163.19,22.48 162.92,22.7
S$12874
  Bottom 0: 162.92,22.7 162.61,22.86
S$12875
  Bottom 0: 162.61,22.86 162.26,22.92
S$12876
  Bottom 0: 162.26,22.92 161.91,22.9
S$12877
  Bottom 0: 161.91,22.9 161.58,22.79
S$12878
  Bottom 0: 161.58,22.79 161.55,22.78
S$12879
  Bottom 0: 161.55,22.78 160.99,23.34
S$12880
  Bottom 0: 160.99,23.34 160.93,23.39
S$12881
  Bottom 0: 160.93,23.39 160.87,23.43
S$12882
  Bottom 0: 160.87,23.43 160.81,23.45
S$12883
  Bottom 0: 160.81,23.45 160.74,23.47
S$12884
  Bottom 0: 160.74,23.47 160.67,23.47
S$12885
  Bottom 0: 160.67,23.47 156.11,23.47
S$12886
  Bottom 0: 156.11,23.47 156.04,23.6
S$12887
  Bottom 0: 156.04,23.6 155.84,23.82
S$12888
  Bottom 0: 155.84,23.82 155.58,23.98
S$12889
  Bottom 0: 155.58,23.98 155.28,24.04
S$12890
  Bottom 0: 155.28,24.04 154.98,24.02
S$12891
  Bottom 0: 154.98,24.02 154.7,23.91
S$12892
  Bottom 0: 154.7,23.91 154.46,23.72
S$12893
  Bottom 0: 154.46,23.72 154.29,23.47
S$12894
  Bottom 0: 154.29,23.47 154.2,23.18
S$12895
  Bottom 0: 154.2,23.18 154.2,22.88
S$12896
  Bottom 0: 154.2,22.88 154.29,22.59
S$12897
  Bottom 0: 154.29,22.59 154.46,22.34
S$12898
  Bottom 0: 154.46,22.34 154.7,22.15
S$12899
  Bottom 0: 154.7,22.15 154.98,22.04
S$12900
  Bottom 0: 154.98,22.04 155.28,22.02
S$12901
  Bottom 0: 155.28,22.02 155.58,22.09
S$12902
  Bottom 0: 155.58,22.09 155.84,22.24
S$12903
  Bottom 0: 155.84,22.24 156.04,22.46
S$12904
  Bottom 0: 156.04,22.46 156.11,22.59
S$12905
  Bottom 0: 156.11,22.59 160.49,22.59
S$12906
  Bottom 0: 160.49,22.59 160.93,22.14
S$12907
  Bottom 0: 160.93,22.14 160.88,22.04
S$12908
  Bottom 0: 160.88,22.04 160.79,21.7
S$12909
  Bottom 0: 160.79,21.7 160.79,21.35
S$12910
  Bottom 0: 160.79,21.35 160.88,21.01
S$12911
  Bottom 0: 160.88,21.01 161.05,20.7
S$12912
  Bottom 0: 161.05,20.7 161.29,20.45
S$12913
  Bottom 0: 161.29,20.45 161.46,20.34
S$12914
  Bottom 0: 161.46,20.34 148.29,20.34
S$12915
  Bottom 0: 164.72,24.32 165.16,24.37
S$12916
  Bottom 0: 165.16,24.37 165.59,24.49
S$12917
  Bottom 0: 165.59,24.49 165.99,24.71
S$12918
  Bottom 0: 165.99,24.71 166.33,24.99
S$12919
  Bottom 0: 166.33,24.99 166.62,25.34
S$12920
  Bottom 0: 166.62,25.34 166.83,25.73
S$12921
  Bottom 0: 166.83,25.73 166.96,26.16
S$12922
  Bottom 0: 166.96,26.16 167,26.61
S$12923
  Bottom 0: 167,26.61 166.96,27.05
S$12924
  Bottom 0: 166.96,27.05 166.83,27.48
S$12925
  Bottom 0: 166.83,27.48 166.62,27.88
S$12926
  Bottom 0: 166.62,27.88 166.33,28.22
S$12927
  Bottom 0: 166.33,28.22 165.99,28.51
S$12928
  Bottom 0: 165.99,28.51 165.59,28.72
S$12929
  Bottom 0: 165.59,28.72 165.16,28.85
S$12930
  Bottom 0: 165.16,28.85 164.72,28.89
S$12931
  Bottom 0: 164.72,28.89 164.27,28.85
S$12932
  Bottom 0: 164.27,28.85 163.84,28.72
S$12933
  Bottom 0: 163.84,28.72 163.45,28.51
S$12934
  Bottom 0: 163.45,28.51 163.1,28.22
S$12935
  Bottom 0: 163.1,28.22 162.82,27.88
S$12936
  Bottom 0: 162.82,27.88 162.6,27.48
S$12937
  Bottom 0: 162.6,27.48 162.47,27.05
S$12938
  Bottom 0: 162.47,27.05 162.43,26.61
S$12939
  Bottom 0: 162.43,26.61 162.47,26.16
S$12940
  Bottom 0: 162.47,26.16 162.6,25.73
S$12941
  Bottom 0: 162.6,25.73 162.82,25.34
S$12942
  Bottom 0: 162.82,25.34 163.1,24.99
S$12943
  Bottom 0: 163.1,24.99 163.45,24.71
S$12944
  Bottom 0: 163.45,24.71 163.84,24.49
S$12945
  Bottom 0: 163.84,24.49 164.27,24.37
S$12946
  Bottom 0: 164.27,24.37 164.72,24.32
S$12947
  Bottom 0: 296.88,21.31 296.91,21.51
S$12948
  Bottom 0: 296.91,21.51 296.87,21.85
S$12949
  Bottom 0: 296.87,21.85 296.74,22.18
S$12950
  Bottom 0: 296.74,22.18 296.53,22.46
S$12951
  Bottom 0: 296.53,22.46 296.26,22.68
S$12952
  Bottom 0: 296.26,22.68 295.95,22.84
S$12953
  Bottom 0: 295.95,22.84 295.6,22.9
S$12954
  Bottom 0: 295.6,22.9 295.25,22.88
S$12955
  Bottom 0: 295.25,22.88 295.14,22.84
S$12956
  Bottom 0: 295.14,22.84 294.84,22.9
S$12957
  Bottom 0: 294.84,22.9 294.49,22.88
S$12958
  Bottom 0: 294.49,22.88 294.16,22.77
S$12959
  Bottom 0: 294.16,22.77 293.87,22.58
S$12960
  Bottom 0: 293.87,22.58 293.63,22.33
S$12961
  Bottom 0: 293.63,22.33 293.45,22.02
S$12962
  Bottom 0: 293.45,22.02 293.43,21.95
S$12963
  Bottom 0: 293.43,21.95 290.27,21.95
S$12964
  Bottom 0: 290.27,21.95 289.52,22.7
S$12965
  Bottom 0: 289.52,22.7 289.54,22.73
S$12966
  Bottom 0: 289.54,22.73 289.58,23.03
S$12967
  Bottom 0: 289.58,23.03 289.54,23.33
S$12968
  Bottom 0: 289.54,23.33 289.4,23.6
S$12969
  Bottom 0: 289.4,23.6 289.2,23.82
S$12970
  Bottom 0: 289.2,23.82 288.94,23.98
S$12971
  Bottom 0: 288.94,23.98 288.64,24.04
S$12972
  Bottom 0: 288.64,24.04 288.34,24.02
S$12973
  Bottom 0: 288.34,24.02 288.06,23.91
S$12974
  Bottom 0: 288.06,23.91 287.86,23.75
S$12975
  Bottom 0: 287.86,23.75 287.86,29.93
S$12976
  Bottom 0: 287.86,29.93 288.06,29.77
S$12977
  Bottom 0: 288.06,29.77 288.34,29.66
S$12978
  Bottom 0: 288.34,29.66 288.64,29.64
S$12979
  Bottom 0: 288.64,29.64 288.94,29.7
S$12980
  Bottom 0: 288.94,29.7 289.2,29.86
S$12981
  Bottom 0: 289.2,29.86 289.4,30.08
S$12982
  Bottom 0: 289.4,30.08 289.54,30.35
S$12983
  Bottom 0: 289.54,30.35 289.58,30.65
S$12984
  Bottom 0: 289.58,30.65 289.54,30.95
S$12985
  Bottom 0: 289.54,30.95 289.4,31.22
S$12986
  Bottom 0: 289.4,31.22 289.2,31.44
S$12987
  Bottom 0: 289.2,31.44 288.94,31.59
S$12988
  Bottom 0: 288.94,31.59 288.64,31.66
S$12989
  Bottom 0: 288.64,31.66 288.34,31.64
S$12990
  Bottom 0: 288.34,31.64 288.06,31.53
S$12991
  Bottom 0: 288.06,31.53 287.86,31.37
S$12992
  Bottom 0: 287.86,31.37 287.86,32.57
S$12993
  Bottom 0: 287.86,32.57 294.88,32.57
S$12994
  Bottom 0: 294.88,32.57 294.88,30.79
S$12995
  Bottom 0: 294.88,30.79 294.89,30.71
S$12996
  Bottom 0: 294.89,30.71 294.93,30.64
S$12997
  Bottom 0: 294.93,30.64 294.99,30.58
S$12998
  Bottom 0: 294.99,30.58 295.06,30.54
S$12999
  Bottom 0: 295.06,30.54 295.13,30.53
S$13000
  Bottom 0: 295.13,30.53 297.54,30.53
S$13001
  Bottom 0: 297.54,30.53 297.62,30.54
S$13002
  Bottom 0: 297.62,30.54 297.69,30.58
S$13003
  Bottom 0: 297.69,30.58 297.75,30.64
S$13004
  Bottom 0: 297.75,30.64 297.79,30.71
S$13005
  Bottom 0: 297.79,30.71 297.8,30.79
S$13006
  Bottom 0: 297.8,30.79 297.8,31.01
S$13007
  Bottom 0: 297.8,31.01 297.82,30.98
S$13008
  Bottom 0: 297.82,30.98 298.06,30.79
S$13009
  Bottom 0: 298.06,30.79 298.34,30.68
S$13010
  Bottom 0: 298.34,30.68 298.64,30.66
S$13011
  Bottom 0: 298.64,30.66 298.76,30.68
S$13012
  Bottom 0: 298.76,30.68 298.85,30.62
S$13013
  Bottom 0: 298.85,30.62 299.16,30.53
S$13014
  Bottom 0: 299.16,30.53 299.49,30.53
S$13015
  Bottom 0: 299.49,30.53 299.8,30.62
S$13016
  Bottom 0: 299.8,30.62 300.07,30.8
S$13017
  Bottom 0: 300.07,30.8 300.17,30.91
S$13018
  Bottom 0: 300.17,30.91 300.17,27.45
S$13019
  Bottom 0: 300.17,27.45 300.16,27.47
S$13020
  Bottom 0: 300.16,27.47 299.95,27.87
S$13021
  Bottom 0: 299.95,27.87 299.67,28.21
S$13022
  Bottom 0: 299.67,28.21 299.32,28.5
S$13023
  Bottom 0: 299.32,28.5 298.92,28.71
S$13024
  Bottom 0: 298.92,28.71 298.5,28.84
S$13025
  Bottom 0: 298.5,28.84 298.05,28.88
S$13026
  Bottom 0: 298.05,28.88 297.67,28.84
S$13027
  Bottom 0: 297.67,28.84 297.29,28.88
S$13028
  Bottom 0: 297.29,28.88 296.84,28.84
S$13029
  Bottom 0: 296.84,28.84 296.42,28.71
S$13030
  Bottom 0: 296.42,28.71 296.02,28.5
S$13031
  Bottom 0: 296.02,28.5 295.67,28.21
S$13032
  Bottom 0: 295.67,28.21 295.39,27.87
S$13033
  Bottom 0: 295.39,27.87 295.17,27.47
S$13034
  Bottom 0: 295.17,27.47 295.05,27.04
S$13035
  Bottom 0: 295.05,27.04 295,26.6
S$13036
  Bottom 0: 295,26.6 295.05,26.15
S$13037
  Bottom 0: 295.05,26.15 295.17,25.72
S$13038
  Bottom 0: 295.17,25.72 295.39,25.33
S$13039
  Bottom 0: 295.39,25.33 295.67,24.98
S$13040
  Bottom 0: 295.67,24.98 296.02,24.7
S$13041
  Bottom 0: 296.02,24.7 296.42,24.48
S$13042
  Bottom 0: 296.42,24.48 296.84,24.36
S$13043
  Bottom 0: 296.84,24.36 297.29,24.31
S$13044
  Bottom 0: 297.29,24.31 297.67,24.35
S$13045
  Bottom 0: 297.67,24.35 298.05,24.31
S$13046
  Bottom 0: 298.05,24.31 298.5,24.36
S$13047
  Bottom 0: 298.5,24.36 298.62,24.39
S$13048
  Bottom 0: 298.62,24.39 297.85,23.63
S$13049
  Bottom 0: 297.85,23.63 297.81,23.57
S$13050
  Bottom 0: 297.81,23.57 297.77,23.52
S$13051
  Bottom 0: 297.77,23.52 297.74,23.45
S$13052
  Bottom 0: 297.74,23.45 297.73,23.39
S$13053
  Bottom 0: 297.73,23.39 297.72,23.32
S$13054
  Bottom 0: 297.72,23.32 297.72,22.15
S$13055
  Bottom 0: 297.72,22.15 296.88,21.31
S$13056
  Bottom 0: 249.09,22.72 249.09,36.12
S$13057
  Bottom 0: 249.09,36.12 249.16,36.17
S$13058
  Bottom 0: 249.16,36.17 249.29,36.38
S$13059
  Bottom 0: 249.29,36.38 249.33,36.63
S$13060
  Bottom 0: 249.33,36.63 249.29,36.88
S$13061
  Bottom 0: 249.29,36.88 249.16,37.09
S$13062
  Bottom 0: 249.16,37.09 249.09,37.14
S$13063
  Bottom 0: 249.09,37.14 249.09,45.73
S$13064
  Bottom 0: 249.09,45.73 257.39,54.04
S$13065
  Bottom 0: 257.39,54.04 257.39,53.83
S$13066
  Bottom 0: 257.39,53.83 257.47,53.52
S$13067
  Bottom 0: 257.47,53.52 257.64,53.24
S$13068
  Bottom 0: 257.64,53.24 257.88,53.02
S$13069
  Bottom 0: 257.88,53.02 258.17,52.87
S$13070
  Bottom 0: 258.17,52.87 258.49,52.8
S$13071
  Bottom 0: 258.49,52.8 258.81,52.82
S$13072
  Bottom 0: 258.81,52.82 259.03,52.9
S$13073
  Bottom 0: 259.03,52.9 260.08,51.85
S$13074
  Bottom 0: 260.08,51.85 260.04,51.83
S$13075
  Bottom 0: 260.04,51.83 259.99,51.77
S$13076
  Bottom 0: 259.99,51.77 259.95,51.7
S$13077
  Bottom 0: 259.95,51.7 259.93,51.63
S$13078
  Bottom 0: 259.93,51.63 259.93,49.85
S$13079
  Bottom 0: 259.93,49.85 259.95,49.77
S$13080
  Bottom 0: 259.95,49.77 259.99,49.7
S$13081
  Bottom 0: 259.99,49.7 260.04,49.64
S$13082
  Bottom 0: 260.04,49.64 260.11,49.6
S$13083
  Bottom 0: 260.11,49.6 260.19,49.59
S$13084
  Bottom 0: 260.19,49.59 261.67,49.59
S$13085
  Bottom 0: 261.67,49.59 257.55,45.47
S$13086
  Bottom 0: 257.55,45.47 257.49,45.4
S$13087
  Bottom 0: 257.49,45.4 257.44,45.33
S$13088
  Bottom 0: 257.44,45.33 257.41,45.24
S$13089
  Bottom 0: 257.41,45.24 257.39,45.16
S$13090
  Bottom 0: 257.39,45.16 257.38,45.07
S$13091
  Bottom 0: 257.38,45.07 257.38,32.75
S$13092
  Bottom 0: 257.38,32.75 257.36,32.78
S$13093
  Bottom 0: 257.36,32.78 257.28,32.82
S$13094
  Bottom 0: 257.28,32.82 257.21,32.83
S$13095
  Bottom 0: 257.21,32.83 255.43,32.83
S$13096
  Bottom 0: 255.43,32.83 255.35,32.82
S$13097
  Bottom 0: 255.35,32.82 255.28,32.78
S$13098
  Bottom 0: 255.28,32.78 255.23,32.72
S$13099
  Bottom 0: 255.23,32.72 255.19,32.65
S$13100
  Bottom 0: 255.19,32.65 255.18,32.58
S$13101
  Bottom 0: 255.18,32.58 255.18,30.8
S$13102
  Bottom 0: 255.18,30.8 255.19,30.72
S$13103
  Bottom 0: 255.19,30.72 255.23,30.65
S$13104
  Bottom 0: 255.23,30.65 255.28,30.59
S$13105
  Bottom 0: 255.28,30.59 255.35,30.55
S$13106
  Bottom 0: 255.35,30.55 255.43,30.54
S$13107
  Bottom 0: 255.43,30.54 256.91,30.54
S$13108
  Bottom 0: 256.91,30.54 249.09,22.72
S$13109
  Bottom 0: 302.95,24.91 302.88,25
S$13110
  Bottom 0: 302.88,25 302.61,25.23
S$13111
  Bottom 0: 302.61,25.23 302.3,25.38
S$13112
  Bottom 0: 302.3,25.38 301.95,25.44
S$13113
  Bottom 0: 301.95,25.44 301.6,25.42
S$13114
  Bottom 0: 301.6,25.42 301.5,25.38
S$13115
  Bottom 0: 301.5,25.38 301.19,25.44
S$13116
  Bottom 0: 301.19,25.44 300.9,25.42
S$13117
  Bottom 0: 300.9,25.42 300.92,25.44
S$13118
  Bottom 0: 300.92,25.44 300.97,25.5
S$13119
  Bottom 0: 300.97,25.5 301,25.55
S$13120
  Bottom 0: 301,25.55 301.03,25.62
S$13121
  Bottom 0: 301.03,25.62 301.05,25.69
S$13122
  Bottom 0: 301.05,25.69 301.05,25.76
S$13123
  Bottom 0: 301.05,25.76 301.05,34.12
S$13124
  Bottom 0: 301.05,34.12 301.22,33.96
S$13125
  Bottom 0: 301.22,33.96 301.34,33.9
S$13126
  Bottom 0: 301.34,33.9 301.34,31.78
S$13127
  Bottom 0: 301.34,31.78 301.35,31.69
S$13128
  Bottom 0: 301.35,31.69 301.37,31.61
S$13129
  Bottom 0: 301.37,31.61 301.4,31.52
S$13130
  Bottom 0: 301.4,31.52 301.45,31.45
S$13131
  Bottom 0: 301.45,31.45 301.51,31.38
S$13132
  Bottom 0: 301.51,31.38 302.95,29.94
S$13133
  Bottom 0: 302.95,29.94 302.95,24.91
S$13134
  Bottom 0: 109.72,25.85 109.81,26.16
S$13135
  Bottom 0: 109.81,26.16 109.86,26.61
S$13136
  Bottom 0: 109.86,26.61 109.81,27.05
S$13137
  Bottom 0: 109.81,27.05 109.69,27.48
S$13138
  Bottom 0: 109.69,27.48 109.47,27.88
S$13139
  Bottom 0: 109.47,27.88 109.19,28.22
S$13140
  Bottom 0: 109.19,28.22 108.84,28.51
S$13141
  Bottom 0: 108.84,28.51 108.44,28.72
S$13142
  Bottom 0: 108.44,28.72 108.02,28.85
S$13143
  Bottom 0: 108.02,28.85 107.57,28.89
S$13144
  Bottom 0: 107.57,28.89 107.12,28.85
S$13145
  Bottom 0: 107.12,28.85 106.7,28.72
S$13146
  Bottom 0: 106.7,28.72 106.3,28.51
S$13147
  Bottom 0: 106.3,28.51 105.96,28.22
S$13148
  Bottom 0: 105.96,28.22 105.67,27.88
S$13149
  Bottom 0: 105.67,27.88 105.46,27.48
S$13150
  Bottom 0: 105.46,27.48 105.33,27.05
S$13151
  Bottom 0: 105.33,27.05 105.29,26.61
S$13152
  Bottom 0: 105.29,26.61 105.33,26.16
S$13153
  Bottom 0: 105.33,26.16 105.42,25.86
S$13154
  Bottom 0: 105.42,25.86 96.63,34.65
S$13155
  Bottom 0: 96.63,34.65 103.89,41.92
S$13156
  Bottom 0: 103.89,41.92 103.95,41.98
S$13157
  Bottom 0: 103.95,41.98 104,42.06
S$13158
  Bottom 0: 104,42.06 104.04,42.14
S$13159
  Bottom 0: 104.04,42.14 104.05,42.23
S$13160
  Bottom 0: 104.05,42.23 104.06,42.32
S$13161
  Bottom 0: 104.06,42.32 104.06,51.79
S$13162
  Bottom 0: 104.06,51.79 114.75,51.79
S$13163
  Bottom 0: 114.75,51.79 114.73,51.77
S$13164
  Bottom 0: 114.73,51.77 114.69,51.7
S$13165
  Bottom 0: 114.69,51.7 114.68,51.63
S$13166
  Bottom 0: 114.68,51.63 114.68,49.85
S$13167
  Bottom 0: 114.68,49.85 114.69,49.77
S$13168
  Bottom 0: 114.69,49.77 114.73,49.7
S$13169
  Bottom 0: 114.73,49.7 114.78,49.64
S$13170
  Bottom 0: 114.78,49.64 114.86,49.6
S$13171
  Bottom 0: 114.86,49.6 114.93,49.59
S$13172
  Bottom 0: 114.93,49.59 116.71,49.59
S$13173
  Bottom 0: 116.71,49.59 116.79,49.6
S$13174
  Bottom 0: 116.79,49.6 116.86,49.64
S$13175
  Bottom 0: 116.86,49.64 116.91,49.7
S$13176
  Bottom 0: 116.91,49.7 116.95,49.77
S$13177
  Bottom 0: 116.95,49.77 116.96,49.85
S$13178
  Bottom 0: 116.96,49.85 116.96,51.63
S$13179
  Bottom 0: 116.96,51.63 116.95,51.7
S$13180
  Bottom 0: 116.95,51.7 116.91,51.77
S$13181
  Bottom 0: 116.91,51.77 116.9,51.79
S$13182
  Bottom 0: 116.9,51.79 117.92,51.79
S$13183
  Bottom 0: 117.92,51.79 117.89,51.78
S$13184
  Bottom 0: 117.89,51.78 117.61,51.6
S$13185
  Bottom 0: 117.61,51.6 117.4,51.36
S$13186
  Bottom 0: 117.4,51.36 117.26,51.06
S$13187
  Bottom 0: 117.26,51.06 117.22,50.74
S$13188
  Bottom 0: 117.22,50.74 117.26,50.42
S$13189
  Bottom 0: 117.26,50.42 117.4,50.11
S$13190
  Bottom 0: 117.4,50.11 117.61,49.87
S$13191
  Bottom 0: 117.61,49.87 117.89,49.7
S$13192
  Bottom 0: 117.89,49.7 118.2,49.6
S$13193
  Bottom 0: 118.2,49.6 118.52,49.6
S$13194
  Bottom 0: 118.52,49.6 118.83,49.7
S$13195
  Bottom 0: 118.83,49.7 119.11,49.87
S$13196
  Bottom 0: 119.11,49.87 119.32,50.11
S$13197
  Bottom 0: 119.32,50.11 119.46,50.42
S$13198
  Bottom 0: 119.46,50.42 119.5,50.74
S$13199
  Bottom 0: 119.5,50.74 119.46,51.06
S$13200
  Bottom 0: 119.46,51.06 119.32,51.36
S$13201
  Bottom 0: 119.32,51.36 119.11,51.6
S$13202
  Bottom 0: 119.11,51.6 118.83,51.78
S$13203
  Bottom 0: 118.83,51.78 118.8,51.79
S$13204
  Bottom 0: 118.8,51.79 119.28,51.79
S$13205
  Bottom 0: 119.28,51.79 119.36,51.79
S$13206
  Bottom 0: 119.36,51.79 119.45,51.81
S$13207
  Bottom 0: 119.45,51.81 119.53,51.85
S$13208
  Bottom 0: 119.53,51.85 119.61,51.89
S$13209
  Bottom 0: 119.61,51.89 119.67,51.95
S$13210
  Bottom 0: 119.67,51.95 120.58,52.85
S$13211
  Bottom 0: 120.58,52.85 120.83,52.8
S$13212
  Bottom 0: 120.83,52.8 121.16,52.82
S$13213
  Bottom 0: 121.16,52.82 121.47,52.93
S$13214
  Bottom 0: 121.47,52.93 121.73,53.12
S$13215
  Bottom 0: 121.73,53.12 121.83,53.24
S$13216
  Bottom 0: 121.83,53.24 121.83,47.49
S$13217
  Bottom 0: 121.83,47.49 119.24,44.91
S$13218
  Bottom 0: 119.24,44.91 119.33,45.21
S$13219
  Bottom 0: 119.33,45.21 119.38,45.66
S$13220
  Bottom 0: 119.38,45.66 119.33,46.1
S$13221
  Bottom 0: 119.33,46.1 119.2,46.53
S$13222
  Bottom 0: 119.2,46.53 118.99,46.93
S$13223
  Bottom 0: 118.99,46.93 118.71,47.27
S$13224
  Bottom 0: 118.71,47.27 118.36,47.56
S$13225
  Bottom 0: 118.36,47.56 117.96,47.77
S$13226
  Bottom 0: 117.96,47.77 117.54,47.89
S$13227
  Bottom 0: 117.54,47.89 117.09,47.94
S$13228
  Bottom 0: 117.09,47.94 116.64,47.89
S$13229
  Bottom 0: 116.64,47.89 116.22,47.77
S$13230
  Bottom 0: 116.22,47.77 115.82,47.56
S$13231
  Bottom 0: 115.82,47.56 115.48,47.27
S$13232
  Bottom 0: 115.48,47.27 115.19,46.93
S$13233
  Bottom 0: 115.19,46.93 114.98,46.53
S$13234
  Bottom 0: 114.98,46.53 114.85,46.1
S$13235
  Bottom 0: 114.85,46.1 114.81,45.66
S$13236
  Bottom 0: 114.81,45.66 114.85,45.21
S$13237
  Bottom 0: 114.85,45.21 114.98,44.78
S$13238
  Bottom 0: 114.98,44.78 115.19,44.39
S$13239
  Bottom 0: 115.19,44.39 115.48,44.04
S$13240
  Bottom 0: 115.48,44.04 115.82,43.76
S$13241
  Bottom 0: 115.82,43.76 116.22,43.54
S$13242
  Bottom 0: 116.22,43.54 116.64,43.42
S$13243
  Bottom 0: 116.64,43.42 117.09,43.37
S$13244
  Bottom 0: 117.09,43.37 117.54,43.42
S$13245
  Bottom 0: 117.54,43.42 117.84,43.5
S$13246
  Bottom 0: 117.84,43.5 116.66,42.32
S$13247
  Bottom 0: 116.66,42.32 116.61,42.27
S$13248
  Bottom 0: 116.61,42.27 116.57,42.21
S$13249
  Bottom 0: 116.57,42.21 116.54,42.15
S$13250
  Bottom 0: 116.54,42.15 116.53,42.08
S$13251
  Bottom 0: 116.53,42.08 116.52,42.01
S$13252
  Bottom 0: 116.52,42.01 116.52,40.9
S$13253
  Bottom 0: 116.52,40.9 115.91,40.3
S$13254
  Bottom 0: 115.91,40.3 115.95,40.58
S$13255
  Bottom 0: 115.95,40.58 115.9,40.92
S$13256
